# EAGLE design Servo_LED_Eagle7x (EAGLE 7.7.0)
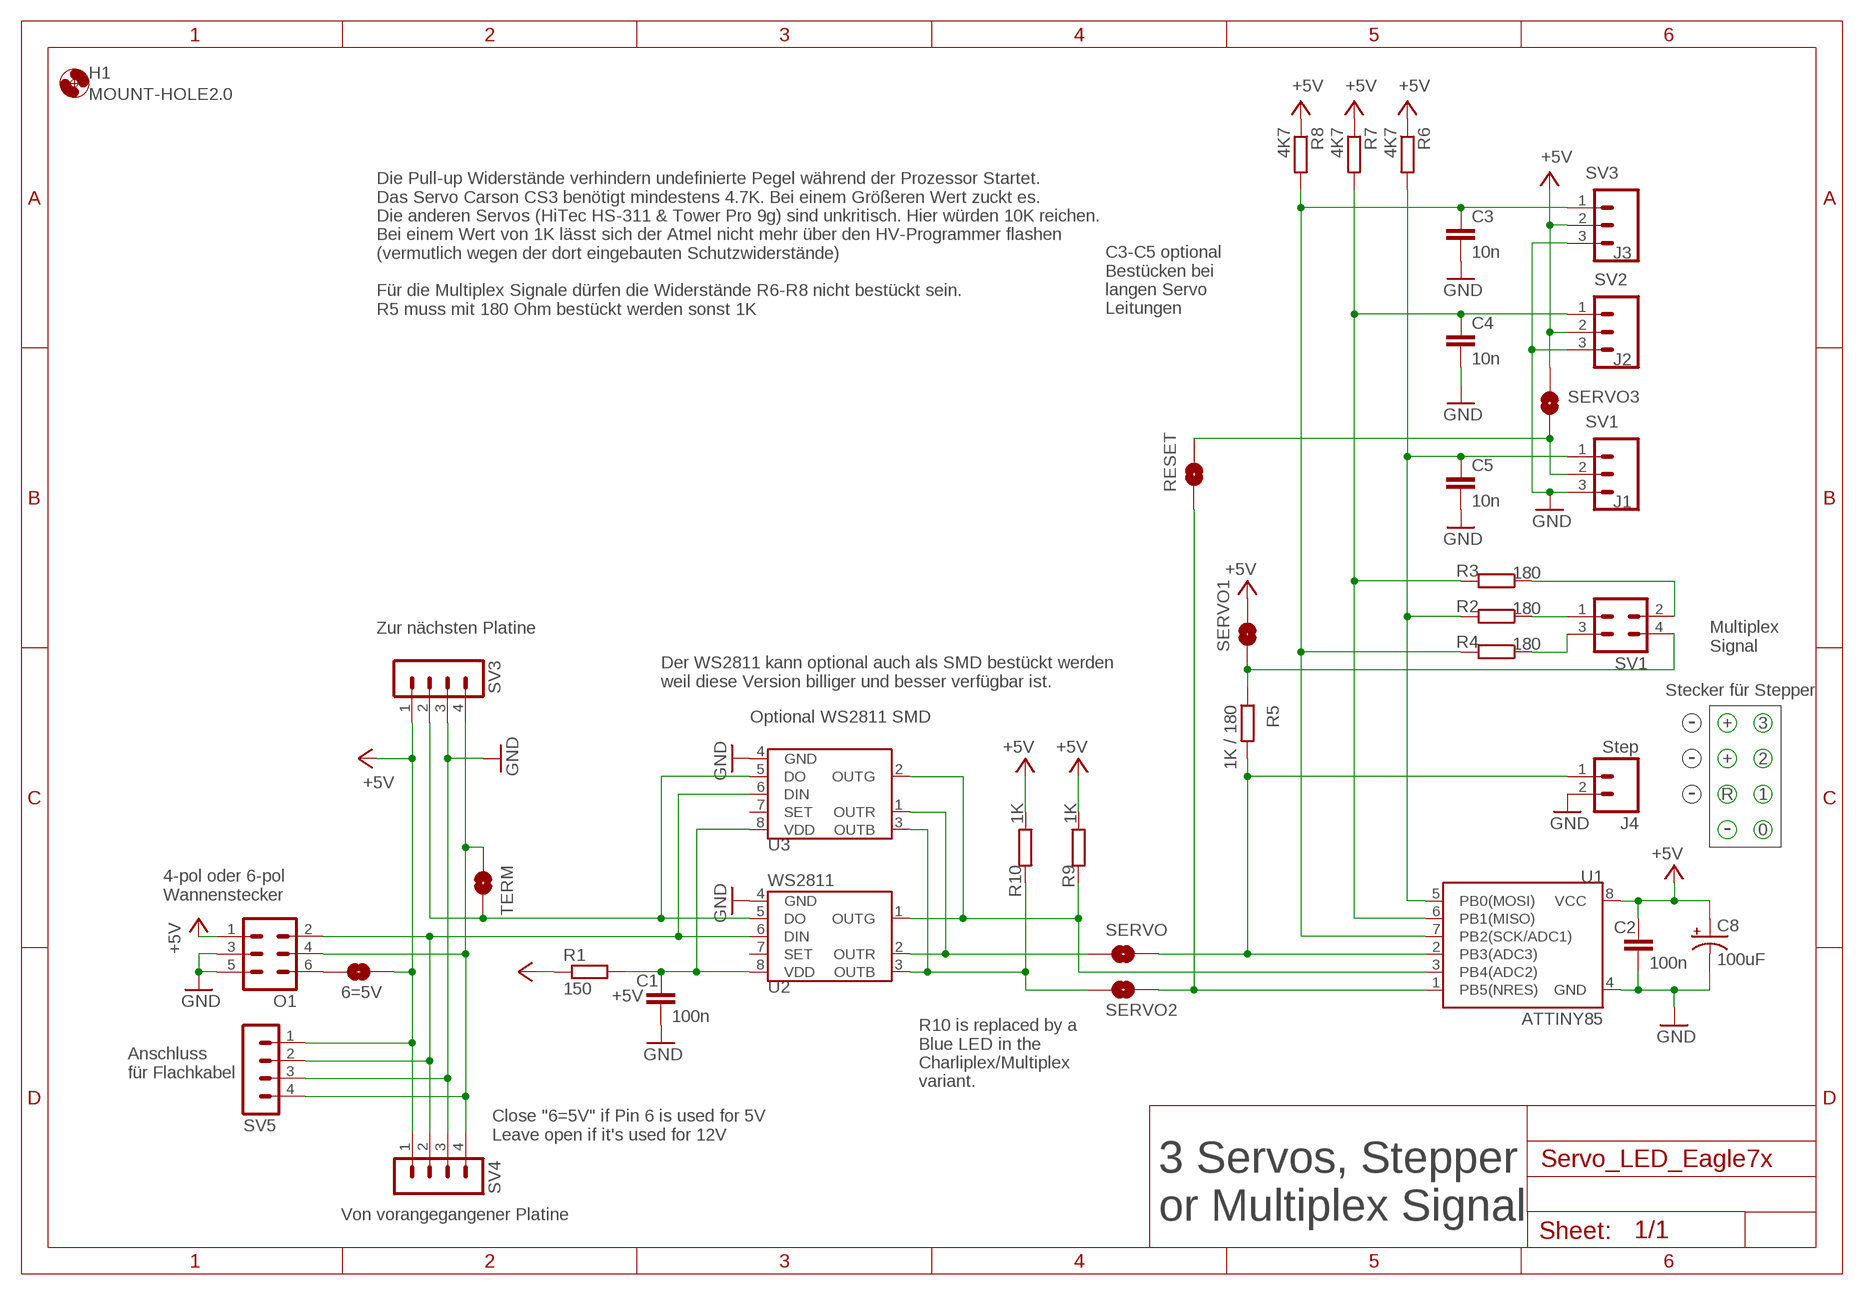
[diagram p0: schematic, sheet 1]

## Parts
6=5V  SOLDERJUMPERNO  [SJ_2S-NO]
C1  100n  C-EU025-024X044  [C025-024X044]
C2  100n  C-EU025-024X044  [C025-024X044]
C3  10n  C-EUC0805  [C0805]
C4  10n  C-EUC0805  [C0805]
C5  10n  C-EUC0805  [C0805]
C8  100uF  SPARKFUN-CAPACITORS_100UF-25V-20%(PTH)  [SPARKFUN-CAPACITORS_CPOL-RADIAL-100UF-25V]
H1  MOUNT-HOLE2.0  [2,0]
J1  SV1  M03PTH  [1X03]
J2  SV2  M03PTH  [1X03]
J3  SV3  M03PTH  [1X03]
J4  Step  M02PTH  [1X02]
O1  ML6  [ML6]
R1  150  RCL_R-EU_0207/2V  [RCL_0207/2V]
R2  180  RCL_R-EU_0207/2V  [RCL_0207/2V]
R3  180  RCL_R-EU_0207/2V  [RCL_0207/2V]
R4  180  RCL_R-EU_0207/2V  [RCL_0207/2V]
R5  1K / 180  RCL_R-EU_0207/2V  [RCL_0207/2V]
R6  4K7  RCL_R-EU_0207/2V  [RCL_0207/2V]
R7  4K7  RCL_R-EU_0207/2V  [RCL_0207/2V]
R8  4K7  RCL_R-EU_0207/2V  [RCL_0207/2V]
R9  1K  RCL_R-EU_0207/2V  [RCL_0207/2V]
R10  1K  RCL_R-EU_0207/2V  [RCL_0207/2V]
RESET  SOLDERJUMPERNO  [SJ_2S-NO]
SERVO  SOLDERJUMPERNO  [SJ_2S-NO]
SERVO1  SOLDERJUMPERNO  [SJ_2S-NO]
SERVO2  SOLDERJUMPERNO  [SJ_2S-NO]
SERVO3  SOLDERJUMPERNO  [SJ_2S-NO]
SV1  MA02-2MUX-SIGNAL  [MUX-SIGNAL]
SV3  MA04-1  [MA04-1]
SV4  MA04-1  [MA04-1]
SV5  MA04-1  [MA04-1]
TERM  SOLDERJUMPERNO  [SJ_2S-NO]
U1  ATTINY85  ATTINY45TINY85-20-DIP  [DIP08]
U2  WS2811  S3PO_MODUL_WS2811_SOUND_MP3-TF-16P_WS2811_AND_ATTINY_WS2811-ICTINY45-20-DIP  [S3PO_MODUL_WS2811_SOUND_MP3-TF-16P_WS2811_AND_ATTINY_WS2811_DIP08]
U3  WS2811 SOT-8  S3PO_MODUL_WS2811_SOUND_MP3-TF-16P_WS2811_AND_ATTINY_WS2811-ICSOP8  [SOP8]

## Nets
+5V: 6=5V.2 C2.1 C8.1(+) J2.2 J3.2 O1.1 R1.1 R6.1 R7.1 R8.1 R9.1 R10.1 SERVO1.2 SERVO3.2 SV3.1 SV4.1 SV5.1 U1.8(VCC)
GND: C1.2 C2.2 C3.2 C4.2 C5.2 C8.2(-) J1.3 J2.3 J3.3 J4.2 O1.3 O1.5 SV3.3 SV4.3 SV5.3 U1.4(GND) U2.4(GND) U3.4(GND)
N$1: O1.2 SV4.2 SV5.2 U2.6(DIN) U3.6(DIN)
N$2: SV3.2 TERM.2 U2.5(DO) U3.5(DO)
N$3: O1.4 SV3.4 SV4.4 SV5.4 TERM.1
N$4: C1.1 R1.2 U2.8(VDD) U3.8(VDD)
N$5: R2.1 SV1.1
N$6: 6=5V.1 O1.6
N$7: R9.2 U1.3(PB4(ADC2)) U2.1(OUTG) U3.2(OUTG)
N$8: J4.1 R5.2 SERVO.2 U1.2(PB3(ADC3))
N$9: C4.1 J2.1 R3.2 R7.2 U1.6(PB1(MISO))
N$10: R4.1 SV1.3
N$11: R3.1 SV1.2
N$12: R5.1 SERVO1.1 SV1.4
N$13: SERVO.1 U2.2(OUTR) U3.1(OUTR)
N$14: C3.1 J3.1 R4.2 R8.2 U1.7(PB2(SCK/ADC1))
N$15: RESET.1 SERVO2.2 U1.1(PB5(NRES))
N$16: C5.1 J1.1 R2.2 R6.2 U1.5(PB0(MOSI))
N$17: J1.2 RESET.2 SERVO3.1
N$18: R10.2 SERVO2.1 U2.3(OUTB) U3.3(OUTB)
Unconnected: U2.7(SET) U3.7(SET)

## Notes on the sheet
- Die Pull-up Widerstände verhindern undefinierte Pegel während der Prozessor Startet. 
  Das Servo Carson CS3 benötigt mindestens 4.7K. Bei einem Größeren Wert zuckt es. 
  Die anderen Servos (HiTec HS-311 & Tower Pro 9g) sind unkritisch. Hier würden 10K reichen. 
  Bei einem Wert von 1K lässt sich der Atmel nicht mehr über den HV-Programmer flashen 
  (vermutlich wegen der dort eingebauten Schutzwiderstände) 
  
  Für die Multiplex Signale dürfen die Widerstände R6-R8 nicht bestückt sein.
  R5 muss mit 180 Ohm bestückt werden sonst 1K
- C3-C5 optional 
  Bestücken bei
  langen Servo 
  Leitungen
- Zur nächsten Platine
- Multiplex
  Signal
- Der WS2811 kann optional auch als SMD bestückt werden
  weil diese Version billiger und besser verfügbar ist.
- Stecker für Stepper
- -
- Optional WS2811 SMD | + | 3
- -
- + | 2
- -
- R | 1
- -
- 0
- 4-pol oder 6-pol 
  Wannenstecker
- Anschluss
  für Flachkabel
- R10 is replaced by a 
  Blue LED in the 
  Charliplex/Multiplex 
  variant.
- Close "6=5V" if Pin 6 is used for 5V
  Leave open if it's used for 12V
- Von vorangegangener Platine
- 3 Servos, Stepper
  or Multiplex Signal

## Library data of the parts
6=5V RESET SERVO SERVO1-SERVO3 TERM = SparkFun-Retired:SOLDERJUMPER: Solder Jumper
C1-C5 = rcl:C-EU: CAPACITOR, European symbol; SPICEPREFIX: C
C8 = Sound_MP3-TF-16P_and_WS2811:SPARKFUN-CAPACITORS_100UF-25V-20%(PTH): CAP-08439; PROD_ID: CAP-08439
H1 = holes:MOUNT-HOLE: MOUNTING HOLE with drill center marker
J1-J3 = SparkFun-Connectors:M03: Header 3 Standard 3-pin 0.1" header. Use with straight break away headers (SKU : PRT-00116), right angle break away headers (PRT-00553), swiss pins (PRT-00743), machine pins (PRT-00117), and female headers (PRT-00115). Molex polarized connector foot print use with SKU : PRT-08232 with associated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
J4 = SparkFun-Connectors:M02: Standard 2-pin 0.1" header. Use with
O1 = con-harting-ml:ML6: HARTING; OC_FARNELL: unknown; OC_NEWARK: unknown
R1-R10 = Sound_MP3-TF-16P_and_WS2811:RCL_R-EU_: RESISTOR, European symbol; SPICEPREFIX: R
SV1 = con-lstb:MA02-2: PIN HEADER
SV3-SV5 = con-lstb:MA04-1: PIN HEADER
U1 = SparkFun-DigitalIC:ATTINY45: Atmel 8-pin 2/4/8kB flash uC; PROD_ID: IC-09445; VALUE: TINY85-20-DIP
U2 = S3PO_Modul_WS2811:S3PO_MODUL_WS2811_SOUND_MP3-TF-16P_WS2811_AND_ATTINY_WS2811-IC: Die Pin nummern im Dokument https://cdn-shop.adafruit.com/datasheets/WS2811.pdf für R und G sind vertauscht ;-(; PROD_ID: IC-09439; VALUE: TINY45-20-DIP
U3 = S3PO_Modul_WS2811:S3PO_MODUL_WS2811_SOUND_MP3-TF-16P_WS2811_AND_ATTINY_WS2811-IC: Die Pin nummern im Dokument https://cdn-shop.adafruit.com/datasheets/WS2811.pdf für R und G sind vertauscht ;-(

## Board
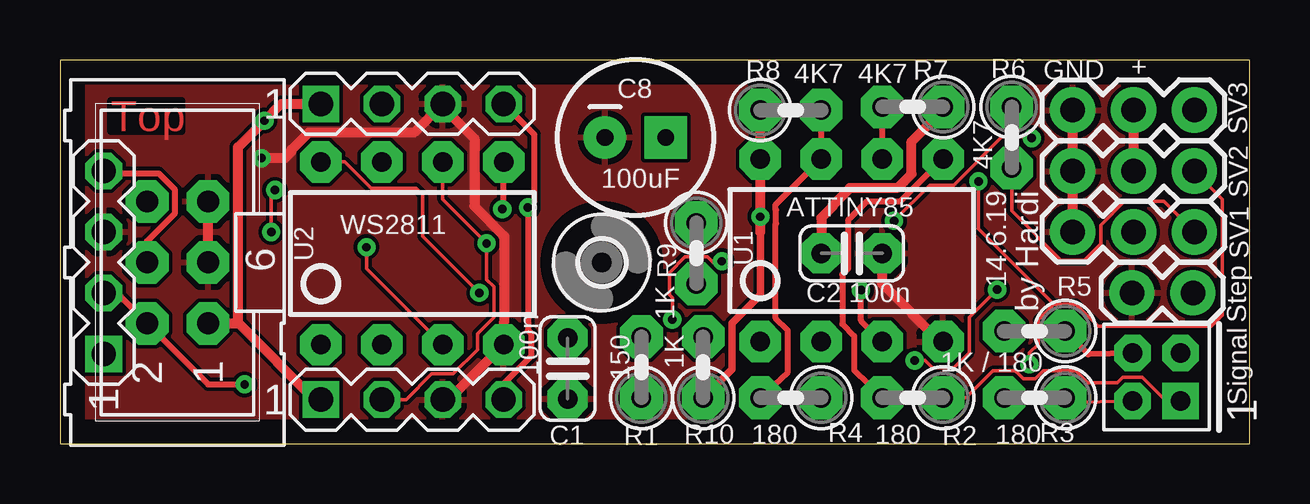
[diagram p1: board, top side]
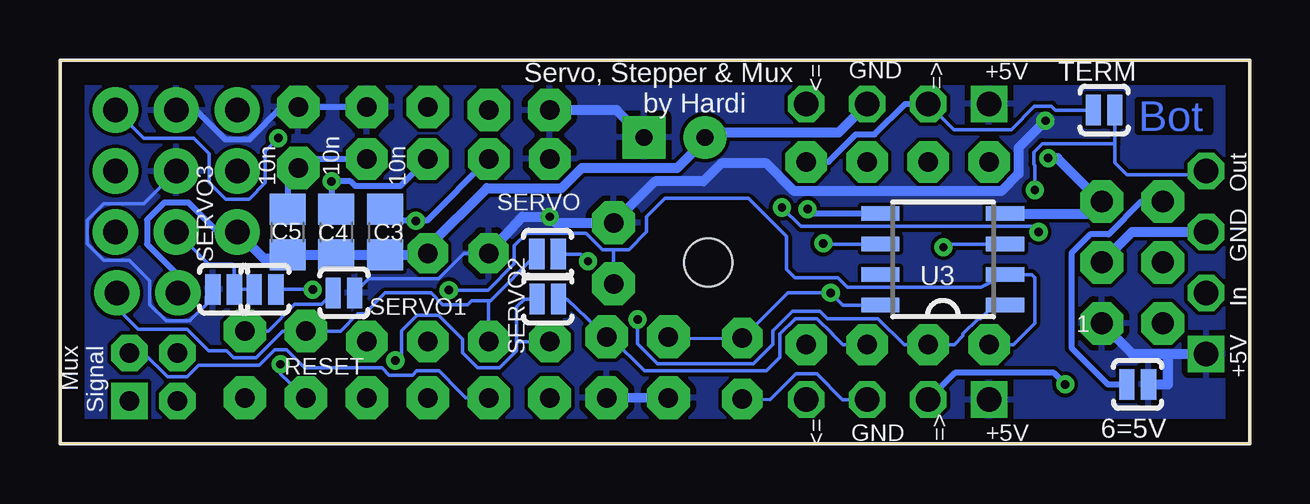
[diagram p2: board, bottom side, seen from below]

Size 49.6 x 15.99 mm. Coordinates in mm from the lower left corner, seen from the top.
Outline: 0,0 49.6,0 49.6,15.99 0,15.99 0,0
Copper layers (1*16): Top 0.035mm / dielectric 1.5mm / Bottom 0.035mm
Design rules "default": minimum track width 6mil, minimum drill 0.35mm, track to track 6mil, track to pad 6mil, pad to pad 6mil, via to via 6mil, smd to smd 6mil, copper to edge 40mil, drill to drill 6mil, minimum pad ring 10mil, minimum via ring 8mil, stop-mask expansion 4mil, vias tented up to drill 0mil, thermal gap 10mil

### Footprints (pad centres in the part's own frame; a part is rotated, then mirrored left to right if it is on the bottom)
SJ_2S-NO = smd 0.635 x 1.27: 1 -0.45,0; 2 0.45,0
C025-024X044 = drill 0.813 pad 1.676 octagon: 1 -1.27,0; 2 1.27,0
C0805 = smd 1.3 x 1.5: 1 -0.95,0; 2 0.95,0
SPARKFUN-CAPACITORS_CPOL-RADIAL-100UF-25V = drill 0.7 pad 1.778 square: 1 1.27,0 | drill 0.7 pad 1.778: 2 -1.27,0
2,0 = hole 2: 0,0
1X03 = drill 1.016 pad 1.88: 1 0,0; 2 2.54,0; 3 5.08,0
1X02 = drill 1.016 pad 1.88: 1 0,0; 2 2.54,0
ML6 = drill 0.914 pad 1.778 octagon: 1 -2.54,-1.27; 2 -2.54,1.27; 3 0,-1.27; 4 0,1.27; 5 2.54,-1.27; 6 2.54,1.27
RCL_0207/2V = drill 0.813 pad 1.778 octagon: 1 -1.27,0; 2 1.27,0
MUX-SIGNAL = drill 0.8 pad 1.524 square: 1 -1,-1 | drill 0.8 pad 1.524 octagon: 2 -1,1; 3 1,-1; 4 1,1
MA04-1 = drill 1.016 pad 1.524 square: 1 -3.81,0 | drill 1.016 pad 1.524 octagon: 2 -1.27,0; 3 1.27,0; 4 3.81,0
DIP08 = drill 0.813 pad 1.727 octagon: 1 -3.81,-3.81; 2 -1.27,-3.81; 3 1.27,-3.81; 4 3.81,-3.81; 5 3.81,3.81; 6 1.27,3.81; 7 -1.27,3.81; 8 -3.81,3.81
S3PO_MODUL_WS2811_SOUND_MP3-TF-16P_WS2811_AND_ATTINY_WS2811_DIP08 = drill 0.813 pad 1.727 octagon: 1 -3.81,-3.81; 2 -1.27,-3.81; 3 1.27,-3.81; 4 3.81,-3.81; 5 3.81,3.81; 6 1.27,3.81; 7 -1.27,3.81; 8 -3.81,3.81
SOP8 = smd 0.6 x 1.6: 1 -1.905,-2.6; 2 -0.635,-2.6; 3 0.635,-2.6; 4 1.905,-2.6; 5 1.905,2.6; 6 0.635,2.6; 7 -0.635,2.6; 8 -1.905,2.6

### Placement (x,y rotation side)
6=5V  4.68,2.48 0 bottom
C1  21.16,3.14 270 top
C2  33,7.94 0 top
C3  36.05,8.83 270 bottom
C4  38.08,8.83 270 bottom
C5  40.11,8.83 270 bottom
C8  23.98,12.76 0 top
H1  22.59,7.55 0 top
J1  47.29,8.83 180 top
J2  47.29,11.37 180 top
J3  47.29,13.91 180 top
J4  47.23,6.28 180 top
O1  4.9,7.55 90 top
R1  24.24,3.19 90 top
R2  35.54,1.92 180 top
R3  40.62,1.92 180 top
R4  30.46,1.92 180 top
R5  40.62,4.7 180 top
R6  39.67,12.76 270 top
R7  35.54,14.03 180 top
R8  30.46,13.91 0 top
R9  26.52,7.94 270 top
R10  26.81,3.19 90 top
RESET  41.05,6.44 180 bottom
SERVO  29.28,7.9 180 bottom
SERVO1  37.76,6.28 0 bottom
SERVO2  29.27,6.03 180 bottom
SERVO3  42.78,6.44 180 bottom
SV1  45.71,2.78 90 top
SV3  14.68,14.16 0 top
SV4  14.68,1.84 0 top
SV5  1.82,7.55 90 top
TERM  6.08,13.91 180 bottom
U1  33,8.06 0 top
U2  14.68,7.94 0 top
U3  12.8,7.68 90 bottom

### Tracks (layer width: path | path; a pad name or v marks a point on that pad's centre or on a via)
+5V  (via drill 0.35)
  Top 0.305: R10.1 26.84,1.95 28,3.11 28,5.01 29.19,6.2 29.19,8.83
  Top 0.406: O1.1 7.44,5.01 | 29.19,8.83 v29.19,9.46 U1.8 R8.1 | C2.1 31.73,9.41 32.21,9.9 32.21,9.94 32.93,10.65 34.91,10.65 35.49,11.24 35.49,12.58 36.81,13.91 R7.1 | J3.2 J2.2 | 7.44,5.01 7.42,5.04 7.42,12.36 v8.52,13.46 9.22,14.16 SV3.1 | 7.44,5.01 10.62,1.84 SV4.1
  Bottom 0.152: C2.1 32.76,7.94 33.83,6.87 36.73,6.87 SERVO1.2 | SERVO3.2 43.52,6.15 43.52,5.8 44.2,5.12 45.17,5.12 45.85,5.8 45.85,6.8 46.71,7.66 47.77,7.66 48.46,8.34 48.46,9.31 47.77,9.99 46.12,9.99 J2.2
  Bottom 0.254: J3.2 43.93,13.91 42.71,12.69 41.7,12.69 40.36,14.03 R6.1 R7.1
  Bottom 0.406: O1.1 4.9,3.75 3.41,3.75 | C8.1 26.4,13.91 R8.1 | C2.1 30.33,9.46 v29.19,9.46 28.94,9.21 R9.1 24.8,10.93 22.78,10.93 22.03,11.68 20.15,11.68 19,10.53 10.37,10.53 9.65,11.24 9.65,12.33 v8.52,13.46 | R1.1 26.75,1.9 R10.1 | 3.41,3.75 SV5.1 | 6=5V.2 3.41,2.48 3.41,3.75
  pour Bottom: 0.71,15.49 49.13,15.49 49.13,0.58 0.71,0.58
GND  (via drill 0.35)
  Top 0.406: O1.3 O1.5 | U1.4 36.68,4.25 34.27,6.67 C2.2 | J1.3 J2.3 J3.3 | SV4.3 16.21,1.84 U2.4 18.49,5.06 18.52,5.08 18.52,8.65 17.27,9.9 17.27,12.71 15.95,14.03 SV3.3 14.76,12.96 10.37,12.96 9.65,12.25 9.65,12.18 9.38,11.9 v8.4,11.9
  Bottom 0.152: SV4.3 16.98,1.84 18.05,2.91 18.93,2.91 20,1.84 C1.2
  Bottom 0.254: J1.3 43.02,8.83 44.24,10.04 45.25,10.04 45.97,9.33 45.97,8.32 44.69,7.04 J4.2
  Bottom 0.406: 6.19,10.07 O1.5 | O1.3 4.9,8.83 SV5.3 | SV3.3 17.15,12.97 22.51,12.97 C8.2 22.71,12.64 23.86,11.49 27.85,11.49 28.69,10.65 31.81,10.65 34.27,8.19 C2.2 34.33,7.88 C3.2 C4.2 C5.2 40.26,7.73 41.11,7.73 J1.3 | v8.4,11.9 8.02,11.9 6.19,10.07 | U3.4 6.68,9.59 6.19,10.07
  pour Top: 0.71,15.49 49.13,15.49 49.13,0.58 0.71,0.58
N$1  (via drill 0.35)
  Top 0.152: SV4.2 14.43,1.84 15.49,2.91 16.39,2.91 17.4,3.91 17.4,4.58 18.09,5.26 18.09,6.54 17.78,6.84 v17.78,8.35 15.95,10.18 U2.6
  Top 0.254: v7.7,2.48 6.17,2.48 O1.2 2.36,6.28 SV5.2
  Bottom 0.152: v17.78,8.35 17.75,8.32 U3.6
  Bottom 0.254: SV4.2 12.29,2.96 8.18,2.96 v7.7,2.48
N$2  (via drill 0.35)
  Top 0.254: v18.44,9.78 18.49,9.83 U2.5
  Bottom 0.152: SV3.2 12.34,13.09 9.95,13.09 8.98,14.07 8.27,14.07 8.11,13.91 TERM.2
  Bottom 0.254: SV3.2 14.37,14.16 15.64,12.89 16.43,12.89 17.57,11.75 U2.5 | U3.5 18.25,9.59 v18.44,9.78
N$3  (via drill 0.35)
  Top 0.152: v8.97,10.58 8.81,10.42 v8.81,8.83
  Top 0.254: O1.4 3.63,8.44 4.8,9.61 4.8,10.58 4.12,11.26 1.92,11.26 SV5.4 | SV4.4 18.49,2.51 19.63,3.65 19.63,4.6 19.51,4.73 v19.51,9.84 19.76,10.1 19.76,12.89 SV3.4
  Bottom 0.152: SV5.4 1.98,11.21 5.13,11.21 5.63,11.71 5.63,12.51 | v8.97,10.58 8.97,11.61 9.01,11.65 9.01,12.15 8.66,12.51 5.63,12.51 | v19.51,9.84 18.72,9.06 9.04,9.06 v8.81,8.83 | TERM.1 5.63,12.51
N$4  (via drill 0.35)
  Top 0.152: U2.8 11.87,11.75 12.96,10.65 14.84,10.65 15.12,10.37 15.12,8.64 v17.48,6.28
  Bottom 0.152: R1.2 24.18,4.38 C1.1 19.25,6.28 v17.48,6.28 16.97,5.78 U3.8
N$5
  Top 0.152: SV1.1 46.11,1.78 45.12,2.77 44.3,2.77 44.07,2.54 42.85,2.54 42.35,3.03 40.98,3.03 40.66,2.71 40.15,2.71 39.87,3 39.85,3 39.81,3.03 38.89,3.03 37.77,1.92 R2.1
N$6
  Bottom 0.254: 6=5V.1 5.92,2.48 7.44,4 7.44,7.94 6.66,8.72 5.89,8.72 4.52,10.1 O1.6
N$7  (via drill 0.35)
  Top 0.254: U1.3 33.39,5.13 v33.39,6.4
  Bottom 0.152: U2.1 9.86,4.13 8.97,5.01 8.97,6.92 9.09,7.05 U3.2 11.21,6.52 16.77,6.52 17.17,6.92 18.97,6.92 19.33,7.28 19.33,8.64 20.91,10.22 24.39,10.22 25.15,9.46 25.15,8.83 25.89,8.09 26.52,8.09 | v33.39,6.4 31.76,6.4 30.66,7.49 30.66,8.24 30.13,8.77 27.67,8.77 26.99,8.09 26.52,8.09 | R9.2 26.52,8.09
N$8
  Bottom 0.152: 31.78,5.97 32.45,5.97 32.62,5.79 33.64,5.79 34.14,6.28 36.04,6.28 36.9,5.42 37.19,5.42 37.91,4.7 R5.2 40.31,4.7 41.43,3.58 42.35,3.58 42.65,3.88 43.4,3.88 44.3,4.77 46.34,4.77 47.23,5.65 J4.1 | U1.2 31.73,5.92 31.78,5.97 | SERVO.2 31.66,5.97 31.78,5.97
N$9  (via drill 0.35)
  Top 0.152: 41.43,5.81 42.35,5.81 43.28,4.89 47.99,4.89 48.46,5.36 48.46,10.2 J2.1 | 41.43,5.81 40.77,5.16 40.77,4.15 40.41,3.78 v40.41,3.31 | 41.43,5.81 38.28,8.96 v38.28,10.93
  Top 0.254: U1.6 R7.2
  Bottom 0.152: v40.41,3.31 40.41,2.89 R3.2
  Bottom 0.254: C4.1 38.28,9.98 v38.28,10.93 37.49,10.93 37.28,10.73 35.41,10.73 U1.6
N$10
  Bottom 0.152: R4.1 32.69,1.92 32.94,2.16 33.81,3.03 34.73,3.03 34.9,2.86 35.87,2.86 36.17,3.16 39.4,3.16 40.15,3.92 40.66,3.92 41.3,3.27 43.81,3.27 44.3,2.79 45.12,2.79 46.11,3.78 SV1.3
N$11
  Top 0.152: SV1.2 42,1.73 R3.1
N$12
  Top 0.254: SV1.4 42.86,3.73 R5.1
  Bottom 0.152: SERVO1.1 38.68,5.81 39.81,5.81 40.93,4.7 R5.1
N$13  (via drill 0.35)
  Top 0.152: v25.52,5.18 25.52,6.09 25.41,6.2 25.41,7.13 26.06,7.78 26.99,7.78 27.22,7.55 27.54,7.55 v27.59,7.61
  Bottom 0.152: U3.1 10.68,5.78 11.24,5.22 11.32,5.22 11.96,4.58 11.96,4.49 12.33,4.13 U2.2 14.41,4.13 15.5,5.22 17.61,5.22 17.91,5.52 19.07,5.52 19.89,4.7 19.89,4.14 20.69,3.34 24.7,3.34 25.53,4.17 25.53,4.84 25.52,4.85 v25.52,5.18 | v27.59,7.61 27.88,7.9 SERVO.1
N$14  (via drill 0.35)
  Top 0.152: v34.76,9.29 36.26,10.78 37.26,10.78 39.27,12.79 40.45,12.79 v40.5,12.73
  Top 0.254: R4.2 30.33,2.98 30.33,4.73 29.83,5.23 29.83,9.17 29.85,9.19 29.85,9.73 29.83,9.76 29.83,9.97 U1.7 R8.2
  Bottom 0.152: v34.76,9.29 34.45,9.29 34.43,9.3 | J3.1 46.12,12.73 44.03,12.73 43.38,12.08 43.38,10.88 42.69,10.2 41.73,10.2 41.04,10.88 41.04,12.2 v40.5,12.73
  Bottom 0.254: U1.7 34.3,9.3 34.43,9.3 36.02,9.3 36.04,9.28 C3.1
N$15  (via drill 0.35)
  Top 0.152: v39.06,6.42 37.9,5.26 37.9,3.8 37.26,3.16 36.36,3.16 36.05,3.47 v35.62,3.47
  Bottom 0.152: RESET.1 39.08,6.44 v39.06,6.42 | v35.62,3.47 35.36,3.73 35.36,4.7 34.72,5.34 33.82,5.34 32.82,4.35 32.82,3.8 32.18,3.16 31.28,3.16 30.56,3.88 30.56,4.25 | SERVO2.2 30.23,6.03 30.56,5.7 30.56,4.25 | U1.1 30.56,4.25
N$16
  Top 0.152: R6.2 39.67,9.71 41.73,7.66 42.69,7.66 43.38,8.34 43.38,9.11 44.37,10.1 46.02,10.1 J1.1
  Top 0.254: R2.2 33.1,3.07 33.1,4.5 32.61,4.99 32.61,7.05 32.85,7.29 32.85,9.31 33.64,10.1 35.03,10.1 U1.5
  Bottom 0.254: U1.5 39.29,11.87 R6.2 40.11,11.05 C5.1
N$17
  Bottom 0.152: RESET.2 SERVO3.1 42.33,7.41 42.4,7.48 43.4,7.48 J1.2
N$18  (via drill 0.35)
  Top 0.152: U2.3 12.78,7.3 v12.78,8.19
  Bottom 0.152: U2.3 16.97,4.13 17.4,4.56 17.4,4.58 18.04,5.22 18.94,5.22 19.58,4.58 19.58,3.6 20.16,3.03 25.24,3.03 26.59,4.38 R10.2 28.46,6.03 SERVO2.1 | v12.78,8.19 12.65,8.32 U3.3

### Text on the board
Top: Top
Bottom: Bot
tPlace: Signal
bPlace: => | <= | +5V | GND | Out | GND | In | +5V | 1 | Mux / Signal | <= | +5V | => | GND
tNames: GND | + | 14.6.19 | by Hardi
bNames: Servo, Stepper & Mux | by Hardi

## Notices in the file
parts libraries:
SparkFun-DigitalIC: Licensing: Creative Commons ShareAlike 4.0 International - https://creativecommons.org/licenses/by-sa/4.0
